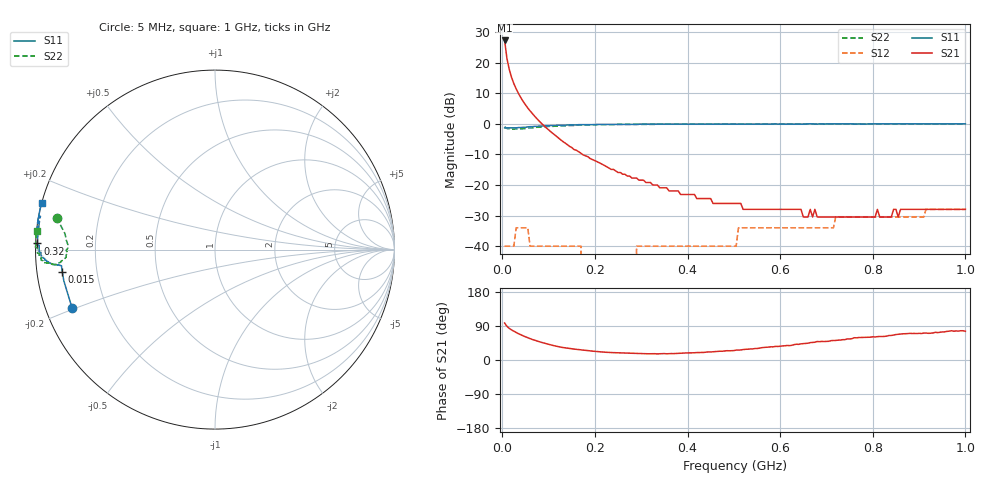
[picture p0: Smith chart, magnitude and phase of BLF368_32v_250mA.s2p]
! Filename:  BLF368_32v_250mA.s2p
! Philips part #: BLF368  !date: 21-05-2003
!32V @250 mA
!D:\Vee measurements\measurement data\VDMOST\BLF368\32v_250mA_#1
# HZ S MA R 50
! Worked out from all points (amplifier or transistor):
!   200 points, 5 MHz to 1 GHz, reference 50 ohm
!   highest |S21| = 27.3 dB at 5 MHz (marker M1)
!   |S21| within 3 dB of that: start of sweep to 7.556 MHz
!   S11 on the Smith chart (normalised r, x): 5 MHz: 0.08, -0.19; 15 MHz: 0.08, -0.07; 320 MHz: 0.01, +0.02; 1 GHz: -0.00, +0.13
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5000000  0.86 -157.9  23.11 97.5  0.01 -2.1  0.9 168.6
1e7  0.86 -168.3  11.76 88.9  0.01 20.9  0.84 174.0
1.5e7  0.86 -171.7  7.79 83.5  0.01 22.3  0.83 176.4
2e7  0.86 -173.1  5.75 79.4  0.01 18.7  0.82 178.1
2.5e7  0.86 -173.7  4.54 76.0  0.01 13.9  0.82 179.5
3e7  0.86 -174.0  3.73 72.5  0.02 8.8  0.83 -179.7
4e7  0.87 -174.3  2.68 66.5  0.02 0.5  0.83 -177.9
5.5e7  0.89 -174.5  1.82 58.8  0.02 -9.6  0.85 -176.0
6e7  0.9 -174.6  1.63 56.4  0.01 -12.3  0.86 -175.7
9.5e7  0.93 -175.6  0.86 42.9  0.01 -25.1  0.9 -174.7
1.7e8  0.97 -178.2  0.33 26.5  0.01 -22.7  0.96 -175.7
1.75e8  0.97 -178.4  0.31 26.0  0 -20.8  0.96 -175.9
2.85e8  0.98 178.7  0.13 17.7  0 66.6  0.98 -178.1
2.9e8  0.98 178.6  0.13 17.3  0.01 68.4  0.98 -178.2
3.2e8  0.99 178.0  0.11 16.5  0.01 75.0  0.98 -178.7
3.4e8  0.99 177.5  0.09 16.5  0.01 76.7  0.99 -178.9
5.05e8  0.99 174.3  0.05 26.2  0.01 88.5  1 178.9
5.1e8  0.99 174.2  0.05 26.2  0.02 88.6  0.99 178.9
6.7e8  1 171.3  0.03 46.3  0.02 90.7  1 177.2
6.75e8  0.99 171.2  0.04 46.9  0.02 90.5  1 177.1
8.35e8  1 168.3  0.03 64.6  0.03 93.3  1 175.7
1e9  1 165.1  0.04 75.8  0.04 92.5  1 173.9
